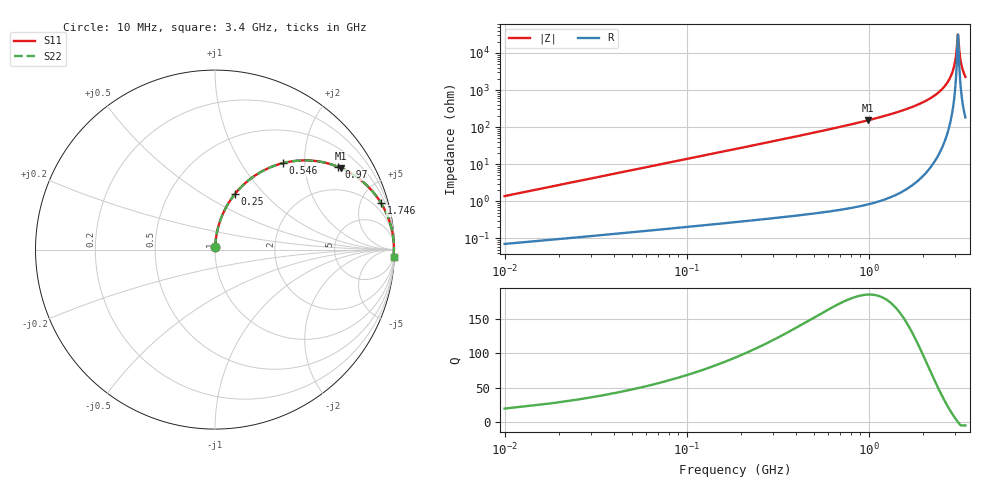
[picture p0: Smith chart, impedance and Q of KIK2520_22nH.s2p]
!version-2
!date-01.2022
!Series
# MHz S RI R 50
!Freq ReS11 ImS11 ReS21 ImS21 ReS12 ImS12 ReS22 ImS22
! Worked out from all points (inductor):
!   425 points, 10 MHz to 3.4 GHz, reference 50 ohm
!   read as one part in series: L = 22 nH near 26 MHz
!   highest Q = 185 at 994 MHz (marker M1), where L = 24.5 nH
!   self-resonance near 3.09 GHz
!   S11 on the Smith chart (normalised r, x): 10 MHz: 1.00, +0.03; 250 MHz: 1.01, +0.70; 546 MHz: 1.01, +1.56; 970 MHz: 1.02, +2.97; 1.746 GHz: 1.06, +7.08; 3.4 GHz: 5, -45
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10  0.000901 0.0138  0.9991 -0.0138  0.9991 -0.0138  0.000901 0.0138
42  0.0047 0.0577  0.9953 -0.0577  0.9953 -0.0577  0.0047 0.0577
82  0.0145 0.1116  0.9855 -0.1116  0.9855 -0.1116  0.0145 0.1116
154  0.0457 0.2031  0.9543 -0.2031  0.9543 -0.2031  0.0457 0.2031
250  0.1102 0.3085  0.8898 -0.3085  0.8898 -0.3085  0.1102 0.3085
546  0.3784 0.4818  0.6216 -0.4818  0.6216 -0.4818  0.3784 0.4818
578  0.4072 0.4882  0.5928 -0.4882  0.5928 -0.4882  0.4072 0.4882
970  0.6876 0.4608  0.3124 -0.4608  0.3124 -0.4608  0.6876 0.4608
994  0.7003 0.4554  0.2997 -0.4554  0.2997 -0.4554  0.7003 0.4554
1146  0.77 0.4181  0.23 -0.4181  0.23 -0.4181  0.77 0.4181
1706  0.9182 0.2704  0.0818 -0.2704  0.0818 -0.2704  0.9182 0.2704
1746  0.9244 0.2605  0.0756 -0.2605  0.0756 -0.2605  0.9244 0.2605
2274  0.9769 0.1426  0.0231 -0.1426  0.0231 -0.1426  0.9769 0.1426
2610  0.9911 0.0791  0.00887 -0.0791  0.00887 -0.0791  0.9911 0.0791
2842  0.9956 0.0395  0.00437 -0.0395  0.00437 -0.0395  0.9956 0.0395
2986  0.9967 0.0166  0.00325 -0.0166  0.00325 -0.0166  0.9967 0.0166
3034  0.9969 0.00915  0.00312 -0.00915  0.00312 -0.00915  0.9969 0.00915
3082  0.9969 0.00186  0.00311 -0.00186  0.00311 -0.00186  0.9969 0.00186
3098  0.9969 -0.000546  0.00312 0.000546  0.00312 0.000546  0.9969 -0.000546
3162  0.9967 -0.01  0.00331 0.01  0.00331 0.01  0.9967 -0.01
3210  0.9964 -0.017  0.00357 0.017  0.00357 0.017  0.9964 -0.017
3400  0.9945 -0.0437  0.00548 0.0437  0.00548 0.0437  0.9945 -0.0437
